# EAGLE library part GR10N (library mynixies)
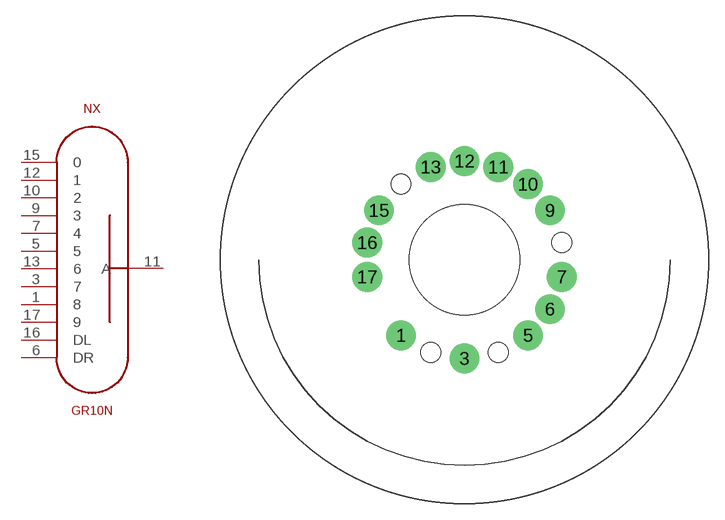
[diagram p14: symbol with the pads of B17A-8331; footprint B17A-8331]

Designator prefix NX

## GR10N  [B17A-8331]
1  8  pas
3  7  pas
5  5  pas
6  DR  pas
7  4  pas
9  3  pas
10  2  pas
11  A  pas
12  1  pas
13  6  pas
15  0  pas
16  DL  pas
17  9  pas

## Footprint B17A-8331 (pad centres in mm)
drill 1.829: 1 -5.861,-6.985; 3 0,-9.119; 5 5.861,-6.985; 6 7.897,-4.559; 7 8.98,-1.583; 9 7.897,4.559; 10 5.861,6.985; 11 3.119,8.569; 12 0,9.119; 13 -3.119,8.569; 15 -7.897,4.559; 16 -8.98,1.583; 17 -8.98,-1.583
hole 1.829 at -3.119,-8.569
hole 1.829 at 3.119,-8.569
hole 1.829 at 8.98,1.583
hole 1.829 at -5.861,6.985
hole 10.16 at 0,0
